(* Logix 5000 Trend export Governer_Operation; software revision 20.01 *)

TYPE Plant :
STRUCT
   Slope_Load : REAL;
   Offset_Efficiency : REAL;
   Actuator_SteadyState : REAL;
   Actuator_Cur : REAL;
   TimeBase : TIMER;
   Actuator_Delta : REAL;
   Speed_Current : DINT;
   Accelleration : DINT;
   Speed_Output : DINT;
   Time_Multiplier : REAL;
   Direct_Frequency_Output : DINT;
   Manual_Actuator_Position : DINT;
   Freq_ComCode : INT;
   Freq_ComCount : INT;
   LoopCounter : COUNTER;
   Act_MTB_Voltage : REAL;
   Feedback_Pos : REAL;
   Update_Outputs : BOOL;
   Chan_Cfg : SINT;
   Speed_Status : SINT;
   Act_Status : SINT;
   Real1 : REAL;
   Real2 : REAL;
   DINT1 : DINT;
   DINT2 : DINT;
END_STRUCT
END_TYPE

TYPE GOVPlus_Input :
STRUCT
   Reserved1 : BOOL;
   Reserved2 : BOOL;
   V3_3Low : BOOL;
   V3_3High : BOOL;
   V5Low : BOOL;
   V5High : BOOL;
   V12_5Low : BOOL;
   V12_5High : BOOL;
   V24Low : BOOL;
   V24High : BOOL;
   AuxLoopLow : BOOL;
   AuxLoopHigh : BOOL;
   Reserved13 : BOOL;
   Reserved14 : BOOL;
   DemandLoopLow : BOOL;
   DemandLoopHigh : BOOL;
   CoolDownInputStatus : BOOL;
   StopInputStatus : BOOL;
   CurrentLoopOutputOpen : BOOL;
   SW1_Enabled_Echo : BOOL;
   SW1_Latching_Echo : BOOL;
   SW1_Failsafe_Echo : BOOL;
   Reserved23 : BOOL;
   Rotating : BOOL;
   AlarmOutActive : BOOL;
   StopOutClosed : BOOL;
   AuxOutputOutOfRange : BOOL;
   Target_Met : BOOL;
   Stop_Echo : BOOL;
   Reserved30 : BOOL;
   VoltOutActive : BOOL;
   V12_5SupplyFaulted : BOOL;
   Breaking : BOOL;
   WatchdogFailure : BOOL;
   FactoryCalEnabled : BOOL;
   WatchdogInhibited : BOOL;
   ActuatorEnabled : BOOL;
   Governing : BOOL;
   Timer1Active : BOOL;
   Timer2Active : BOOL;
   Timer3Active : BOOL;
   Purging : BOOL;
   Cooldown : BOOL;
   Max_Authority : BOOL;
   Demand_Active : BOOL;
   Target_Active : BOOL;
   Voltage_Driver_Output_On : BOOL;
   Reserved48 : BOOL;
   Aux_Output_Alarm : BOOL;
   Actuator_Output_Fault : BOOL;
   Overspeed : BOOL;
   Underspeed : BOOL;
   Stopped : BOOL;
   Reserved54 : BOOL;
   Reserved55 : BOOL;
   Reserved56 : BOOL;
   Reserved57 : BOOL;
   Reserved58 : BOOL;
   Reserved59 : BOOL;
   Reserved60 : BOOL;
   Reserved61 : BOOL;
   Reserved62 : BOOL;
   Reserved63 : BOOL;
   Reserved64 : BOOL;
   GovTime : REAL;
   Accelleration : REAL;
   RPM : DINT;
   RPMUnfiltered : REAL;
   DemandInput : REAL;
   AuxInput : REAL;
   CurrentOut : REAL;
   VoltageOut : REAL;
   Voltage_240 : REAL;
   Voltage_100 : REAL;
   Voltage_50 : REAL;
   Voltage_33 : REAL;
   Voltage_Output_Sense_Value : REAL;
   DemandTarget : DINT;
   ProcessorUsage : INT;
   GovState : INT;
   Speed_Target : REAL;
   Acceleration_Target : REAL;
   Acceleration_Error : REAL;
   RPM_Error : INT;
   Actuator_Position_Output : INT;
   ActuatorCounts : DINT;
   UpWindow : INT;
   DownWindow : INT;
   Float_Rsp : REAL;
   Comm_Status : INT;
   Spare_Echo : INT;
   Aux_Out_Echo : REAL;
END_STRUCT
END_TYPE

VAR_GLOBAL   (* controller tags *)
   GOV_Input : GOVPlus_Input := (SW1_Enabled_Echo := 1, SW1_Latching_Echo := 1, SW1_Failsafe_Echo := 1, Rotating := 1, StopOutClosed := 1, Target_Met := 1, Stop_Echo := 1, VoltOutActive := 1, WatchdogFailure := 1, ActuatorEnabled := 1, Governing := 1, Timer1Active := 1, Timer2Active := 1, Timer3Active := 1, Demand_Active := 1, Target_Active := 1, GovTime := 9.899902, Accelleration := -19.989746, RPM := 433, RPMUnfiltered := 413.57422, DemandInput := 18.0, AuxInput := 4.959961, CurrentOut := 5.329956, VoltageOut := 9.98999, Voltage_240 := 22.899902, Voltage_100 := 12.399902, Voltage_50 := 5.2999268, Voltage_33 := 3.1999512, Voltage_Output_Sense_Value := 9.899902, DemandTarget := 1800, ProcessorUsage := 37, GovState := 10, Speed_Target := 400.0, Acceleration_Target := -35.029297, Acceleration_Error := 15.039795, RPM_Error := 13, Actuator_Position_Output := 8, ActuatorCounts := 4276, UpWindow := 5, DownWindow := 5, Float_Rsp := 2.3999634, Comm_Status := 523, Aux_Out_Echo := 10.0);
   GOVPlus_Simulator : Plant := (Slope_Load := 15.0, Offset_Efficiency := 25.0, Actuator_SteadyState := 7380.0, Actuator_Cur := 6170.0, TimeBase.PRE := 100, Actuator_Delta := -1210.0, Speed_Current := 467, Accelleration := -81, Speed_Output := 459, Time_Multiplier := 0.1, Direct_Frequency_Output := 25, Manual_Actuator_Position := 4095, Act_MTB_Voltage := 9.88, Feedback_Pos := -24.9375, Update_Outputs := 1, Chan_Cfg := 2);
END_VAR

TREND Governer_Operation (sample period 100 ms) : GOVPlus_Simulator.Slope_Load, GOVPlus_Simulator.Actuator_Cur, GOVPlus_Simulator.Speed_Current, GOV_Input.Speed_Target
